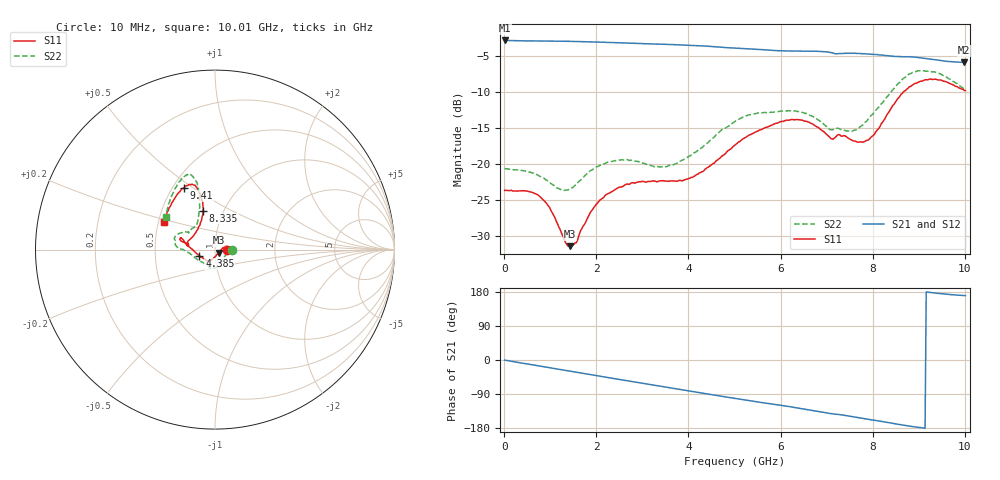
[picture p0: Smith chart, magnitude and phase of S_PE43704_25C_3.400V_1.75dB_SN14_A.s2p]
! Device ID: PE43704
! Dir: z:\PE43704\PE43704_Char_1_20130516\PE43704\AMB\3p400V\1p75dB
! Serial: 14
! Insertion: A
! Impedance: 50 ohm
! Temp: Amb
! VDD: 3.400V
! Attenuation Step: 1.75dB
! IDD: 1.140365e-01mA
#  Hz  S  RI  R  50
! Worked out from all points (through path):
!   401 points, 10 MHz to 10.01 GHz, reference 50 ohm
!   highest |S21| = -2.80 dB at 10 MHz (marker M1); lowest = -5.8 dB at 9.985 GHz (marker M2)
!   group delay of S21, straight-line fit = 54 ps
!   lowest |S11| = -31.4 dB at 1.435 GHz (marker M3), VSWR 1.06, Z = 52.1 - j1.79 ohm
!   |S11| at or under -10 dB: start of sweep to 8.659 GHz
!   |S22| runs from -23.6 to -7.0 dB; largest |S21 - S12| = 0.0051
!   S11 on the Smith chart (normalised r, x): 10 MHz: 1.14, +0.00; 4.385 GHz: 0.84, -0.06; 8.335 GHz: 0.80, +0.37; 9.41 GHz: 0.57, +0.46; 10.01 GHz: 0.53, +0.18
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1e7  0.0657 0.000216  0.7244 -0.00294  0.7243 -0.00287  0.0932 1.89e-05
7.6e8  0.0565 0.0207  0.6916 -0.1941  0.6916 -0.1941  0.0829 0.0047
1.435e9  0.0208 -0.0172  0.6209 -0.3525  0.6207 -0.3526  0.047 -0.0482
1.685e9  0.00515 -0.0352  0.5843 -0.4058  0.5844 -0.4058  0.0307 -0.0726
1.935e9  -0.00805 -0.0487  0.5427 -0.4539  0.543 -0.4539  0.0156 -0.0911
2.235e9  -0.0204 -0.0585  0.4879 -0.5053  0.4883 -0.505  -0.00113 -0.1026
2.71e9  -0.0332 -0.0643  0.3922 -0.5729  0.3926 -0.5726  -0.0244 -0.1033
3.36e9  -0.0391 -0.0655  0.2502 -0.6355  0.2508 -0.6352  -0.0443 -0.0851
3.91e9  -0.0572 -0.0524  0.1218 -0.6616  0.1225 -0.6616  -0.0899 -0.0605
4.385e9  -0.0865 -0.0352  0.00963 -0.6614  0.0101 -0.6613  -0.1361 -0.0249
5.01e9  -0.1354 0.00821  -0.1257 -0.6288  -0.1256 -0.6291  -0.1979 0.00575
6.035e9  -0.1883 0.0636  -0.3081 -0.5308  -0.3063 -0.5319  -0.2263 0.0598
6.685e9  -0.1855 0.0459  -0.4147 -0.4471  -0.4152 -0.4463  -0.195 0.0915
7.085e9  -0.1482 0.0306  -0.4666 -0.3737  -0.4685 -0.3744  -0.1465 0.0931
7.585e9  -0.1284 0.0676  -0.5118 -0.294  -0.511 -0.2936  -0.1047 0.136
7.935e9  -0.0938 0.1176  -0.5364 -0.2263  -0.5373 -0.2277  -0.0914 0.1917
8.335e9  -0.0662 0.2167  -0.548 -0.1458  -0.5465 -0.1495  -0.086 0.2866
8.36e9  -0.0658 0.2238  -0.548 -0.1407  -0.5474 -0.144  -0.0859 0.2951
8.86e9  -0.099 0.3414  -0.5544 -0.0427  -0.5506 -0.0442  -0.1301 0.4143
9.41e9  -0.1725 0.3444  -0.5278 0.038  -0.527 0.0391  -0.1927 0.3835
9.985e9  -0.2804 0.166  -0.5026 0.0881  -0.5046 0.0898  -0.2718 0.1884
1.001e10  -0.2854 0.1539  -0.504 0.09  -0.5066 0.0904  -0.2744 0.1792
